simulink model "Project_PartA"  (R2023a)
settings: Solver=FixedStepAuto  StartTime=0.0  StopTime=inf  FixedStep=.01  RelTol=1e-3  EnableMultiTasking=on
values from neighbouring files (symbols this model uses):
  encoderResolution = 48    [project_constants.m]
  gearRatio = 171.79    [project_constants.m]
libraries: arduinolib x2, arduinosensorlib x1

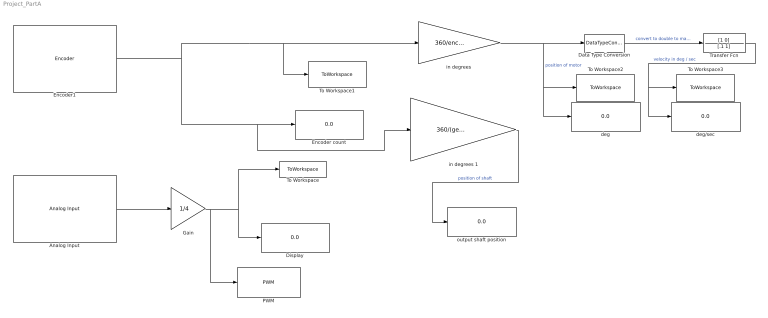
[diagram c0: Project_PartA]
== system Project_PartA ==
  Analog Input : arduinolib/Analog Input  pinNumber=0  ReadResultsOnly=off  ConversionTriggerSource=Software  ExternalTriggerType=uint32( 0 )  OutputDataType=uint16  EnableConversionCompleteNotify=off  EnableOuputStatus=off  SampleTime=-1  blockPlatform=arduino
  Data Type Conversion : DataTypeConversion  OutDataTypeStr=double
  Display : Display
  Encoder count : Display
  Encoder1 : arduinosensorlib/Encoder  InputA=2  InputB=3  Mode=No reset  SampleTime=-1
  Gain : Gain  Gain=1/4
  PWM : arduinolib/PWM  pinNumber=9  frequencyType=Default  desiredFrequency=490.2  achievableFrequency=490.2
  To Workspace : ToWorkspace  VariableName=pot_reading  SaveFormat=Structure With Time  SampleTime=-1
  To Workspace1 : ToWorkspace  VariableName=encoder_reading  SaveFormat=Structure With Time  SampleTime=-1
  To Workspace2 : ToWorkspace  VariableName=position  SaveFormat=Structure With Time  SampleTime=-1
  To Workspace3 : ToWorkspace  VariableName=speed  SaveFormat=Structure With Time  SampleTime=-1
  Transfer Fcn : TransferFcn  Numerator=[1 0]  Denominator=[.1 1]
  deg : Display
  deg/sec : Display
  "in degrees " : Gain  Gain=360/encoderResolution
  in degrees 1 : Gain  Gain=360/(gearRatio*encoderResolution)
  output shaft position : Display
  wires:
  Analog Input/1 -> Gain/1
  Gain/1 -> PWM/1, To Workspace/1, Display/1
  Encoder1/1 -> "in degrees "/1, To Workspace1/1, in degrees 1/1, Encoder count/1
  Transfer Fcn/1 -> deg/sec/1, To Workspace3/1  "velocity in deg / sec"
  Data Type Conversion/1 -> Transfer Fcn/1  "convert to double to make TF happy"
  "in degrees "/1 -> Data Type Conversion/1, deg/1, To Workspace2/1  "position of motor"
  in degrees 1/1 -> output shaft position/1  "position of shaft"
